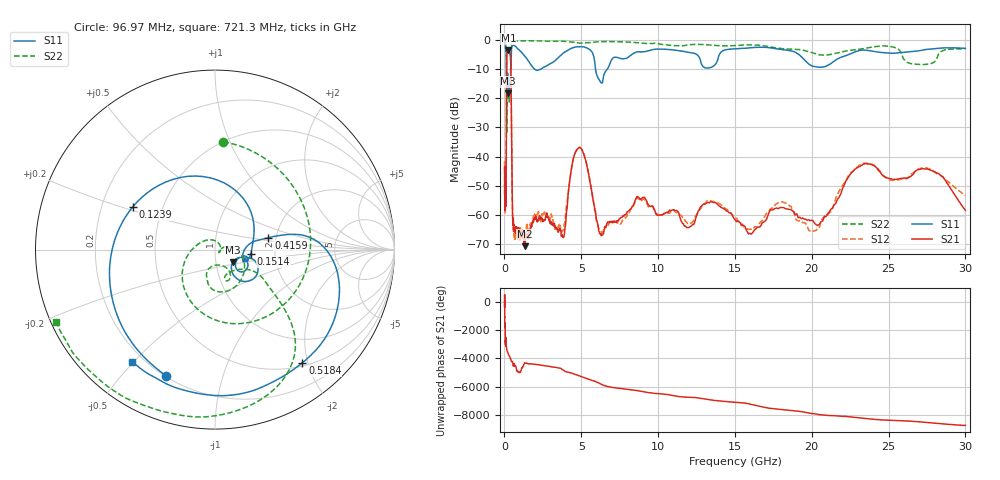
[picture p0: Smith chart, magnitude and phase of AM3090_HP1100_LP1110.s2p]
! Date/Time: Thu, Feb 28, 2019 2:07 PM
! Network Analyzer: Agilent Technologies E8364B Rev: A.07.50.67
! Sweep from 0.010 to 30.000 GHz, 1601 Points, Sweep Type: LOG
! Power Supply: 5.022 V, 0.002 A
# Hz S DB R 50
!freq MagS11 AngS11 MagS21 AngS21 MagS12 AngS12 MagS22 AngS22
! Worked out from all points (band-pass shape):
!   1601 points, 10 MHz to 30 GHz, reference 50 ohm
!   highest |S21| = -3.62 dB at 253.4 MHz (marker M1); lowest = -70.6 dB at 1.315 GHz (marker M2)
!   |S21| within 3 dB of the highest: 144.8 MHz to 399.8 MHz (255.1 MHz wide, 93.7 % of centre)
!   lowest |S11| = -18.3 dB at 246 MHz (marker M3), VSWR 1.28, Z = 60.4 - j8.57 ohm
!   |S11| at or under -10 dB: 136.1 MHz to 417.9 MHz (281.8 MHz wide, 102 % of centre); 1.972 GHz to 2.384 GHz (412.2 MHz wide, 18.9 % of centre); 5.926 GHz to 6.696 GHz (769.8 MHz wide, 12.2 % of centre)
!   |S22| runs from -32.0 to -0.2 dB; largest |S21 - S12| = 0.014
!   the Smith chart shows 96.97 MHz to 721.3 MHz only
!   S11 on the Smith chart (normalised r, x): 96.97 MHz: 0.20, -0.67; 123.9 MHz: 0.34, +0.22; 151.4 MHz: 1.50, -0.08; 415.9 MHz: 1.82, +0.27; 518.4 MHz: 0.55, -1.91; 721.3 MHz: 0.16, -0.49
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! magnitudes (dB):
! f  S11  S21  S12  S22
! 10 MHz  -0.3  -44.3  -42.4  -0.7
! 38.04 MHz  -0.4  -55.9  -56.5  -1.5
! 96.97 MHz  -2.4  -55.2  -53.8  -4.4
! 108.8 MHz  -3.5  -49.9  -51.4  -5.1
! 123.9 MHz  -5.7  -27.7  -27.5  -6.4
! 144.7 MHz  -13.3  -6.6  -6.6  -28.0
! 151.4 MHz  -13.9  -5.5  -5.4  -30.6
! 246 MHz  -18.3  -3.6  -3.6  -14.3
! 253.4 MHz  -17.8  -3.6  -3.6  -14.8
! 415.9 MHz  -10.3  -9.2  -9.2  -7.3
! 518.4 MHz  -2.0  -58.0  -56.6  -0.5
! 550.5 MHz  -1.9  -63.7  -62.6  -0.4
! 721.3 MHz  -2.2  -65.3  -67.2  -0.2
! 1.315 GHz  -5.5  -70.6  -68.8  -0.3
! 2.084 GHz  -10.4  -61.1  -60.4  -0.3
! 3.817 GHz  -4.6  -67.5  -65.1  -0.4
! 4.878 GHz  -2.3  -36.9  -36.8  -1.1
! 6.234 GHz  -14.2  -66.5  -65.5  -0.6
! 7.926 GHz  -6.3  -59.6  -60.6  -0.7
! 19.9 GHz  -8.6  -61.9  -65.5  -4.2
! 23.48 GHz  -3.5  -42.4  -42.2  -2.9
! 30 GHz  -2.9  -58.4  -53.3  -3.0
